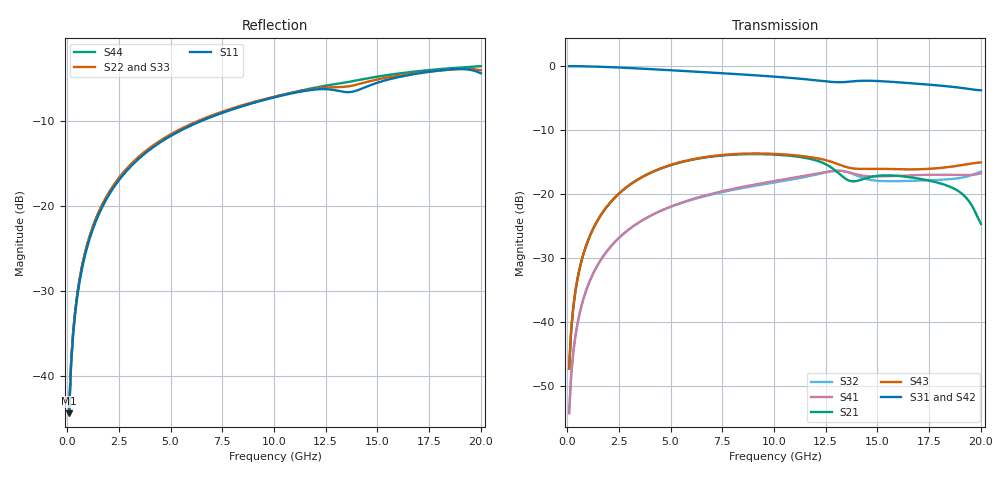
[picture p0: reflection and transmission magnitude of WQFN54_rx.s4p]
! Generated by program util_convert_matmxmd4pspars_to_s4psended on 05-13-2014 07:49:05
!  1 ----xxxxxxxxxxxxxxxxxx---- 3
!  xxxxxxxxxxxxxxxxxx
!  (Input) xxxxxxxxxxxxxxxxxx  (Output)
!  xxxxxxxxxxxxxxxxxx
!  2 ----xxxxxxxxxxxxxxxxxx---- 4
# MHZ S DB R 50.00
! FREQ  S11  S12  S13  S14
!  S21  S22  S23  S24
!  S31  S32  S33  S34
!  S41  S42  S43  S44
!  DB  ANG  DB  ANG  DB  ANG  DB  ANG
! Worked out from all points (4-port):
!   200 points, 100 MHz to 20 GHz, reference 50 ohm
!   strongest paths, dB at 100 MHz, 5.1 GHz, 10.1 GHz, 15.1 GHz, 20 GHz:
!     S31: 0.0, -0.7, -1.7, -2.3, -3.8
!     S42: 0.0, -0.7, -1.7, -2.6, -3.7
!     S43: -47.2, -15.3, -13.7, -16.0, -15.0
!     S21: -47.2, -15.4, -13.8, -17.1, -24.6
!     S41: -54.2, -21.8, -17.9, -17.2, -16.8
!     S32: -54.2, -21.9, -18.1, -17.9, -16.5
!   lowest |S11| = -44.4 dB at 100 MHz (marker M1), VSWR 1.01, Z = 50.1 + j0.594 ohm
!   |S11| at or under -10 dB: start of sweep to 6.447 GHz
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100  -44.36 78.5  -47.17 82.9  -0.01 -0.8  -54.19 -98.7
     -47.17 82.9  -44.02 77.1  -54.16 -99.2  -0.02 -0.9
     -0.01 -0.8  -54.16 -99.2  -44.37 79.3  -47.20 83.1
     -54.19 -98.7  -0.02 -0.9  -47.20 83.1  -44.02 77.7
400  -32.47 83.0  -35.19 83.8  -0.02 -3.3  -42.22 -99.2
     -35.19 83.8  -32.17 82.4  -42.20 -99.1  -0.02 -3.6
     -0.02 -3.3  -42.20 -99.1  -32.46 84.0  -35.22 84.3
     -42.22 -99.2  -0.02 -3.6  -35.22 84.3  -32.16 83.3
1200  -23.02 76.1  -25.79 75.4  -0.07 -9.9  -32.80 -112.9
      -25.79 75.4  -22.73 75.2  -32.78 -112.4  -0.07 -10.6
      -0.07 -9.9  -32.78 -112.4  -23.02 78.8  -25.82 76.9
      -32.80 -112.9  -0.07 -10.6  -25.82 76.9  -22.74 77.6
4700  -12.18 43.1  -15.79 39.7  -0.59 -36.6  -22.33 -171.6
      -15.79 39.7  -11.98 40.5  -22.37 -169.8  -0.64 -39.3
      -0.59 -36.6  -22.37 -169.8  -12.19 53.5  -15.76 45.6
      -22.33 -171.6  -0.64 -39.3  -15.76 45.6  -12.09 50.5
11100  -6.60 -5.5  -14.12 -9.9  -1.93 -80.1  -17.33 100.3
       -14.12 -9.9  -6.54 -8.9  -17.56 102.5  -1.90 -85.7
       -1.93 -80.1  -17.56 102.5  -6.48 16.7  -13.95 7.6
       -17.33 100.3  -1.90 -85.7  -13.95 7.6  -6.50 12.7
18400  -3.92 -45.5  -18.69 -25.4  -3.16 -124.2  -16.96 14.3
       -18.69 -25.4  -3.95 -51.2  -17.67 14.5  -3.30 -133.5
       -3.16 -124.2  -17.67 14.5  -3.91 -20.6  -15.77 17.1
       -16.96 14.3  -3.30 -133.5  -15.77 17.1  -3.78 -30.7
20000  -4.35 -56.5  -24.63 -18.3  -3.77 -131.5  -16.75 1.5
       -24.63 -18.3  -4.00 -61.0  -16.47 -2.0  -3.69 -143.3
       -3.77 -131.5  -16.47 -2.0  -3.69 -30.5  -15.03 19.0
       -16.75 1.5  -3.69 -143.3  -15.03 19.0  -3.52 -40.7
